| IBIS file stm32u595_599_5a5_5a9_lqfp144_smps.ibs
[IBIS ver] 4.2
[File name] stm32u595_599_5a5_5a9_lqfp144_smps.ibs
[File Rev] rev2.1
[Date]  11-09-2023
[Source] Data Created at STMicroelectronics
[Notes]  File originated from ELDO simulations.
[Disclaimer]  This information is for modeling purpose only and is
   not guaranteed. The information is subject to change without
   notice.
[Copyright] Copyright 2023 STMicroelectronics Inc.
|   Component stm32u595_599_5a5_5a9_lqfp144_smps
[Component] stm32u595_599_5a5_5a9_lqfp144_smps
[Manufacturer] STMicroelectronics
[Package]
| variable   typ   min   max
R_pkg  0  NA  NA
L_pkg  0  NA  NA
C_pkg  0  NA  NA
[Pin]   signal_name   model_name
1  PE2  io8_100m_hslv_ft
2  PE3  io8_100m_hslv_tamp_ft
3  PE4  io8_100m_hslv_tamp_ft
4  PE5  io8_100m_hslv_tamp_ft
5  PE6  io8_100m_hslv_tamp_ft
6  VBAT  power
7  PC13  io8_100m_ft
8  PC14-OSC32_IN  nc
9  PC15-OSC32_OUT  nc
10  PF0  io8_100m_hslv_ft
11  PF1  io8_100m_hslv_ft
12  PF2  io8_100m_hslv_ft
13  PF3  io8_100m_hslv_ft
14  PF4  io8_100m_i2c_ft
15  PF5  io8_100m_i2c_ft
16  VSS  gnd
17  VDD  power
18  PF6  io8_100m_hslv_ft
19  PF7  io8_100m_hslv_ft
20  PF8  io8_100m_hslv_ft
21  PF9  io8_100m_hslv_ft
22  PF10  io8_166m_hslv_ft
23  PH0-OSC_IN  nc
24  PH1-OSC_OUT  nc
25  NRST  nc
26  PC0  io8_100m_hslv_ft
27  PC1  io8_spi_hslv_ft
28  PC2  io8_100m_hslv_ft
29  PC3  io8_100m_hslv_ft
30  VSSA  nc
31  VREFP  nc
32  VDDA  nc
33  PA0  io8_100m_hslv_tamp_ft
34  PA1  io8_100m_hslv_tamp_ft
35  PA2  io8_100m_hslv_ft
36  PA3  io8_166m_hslv_ft
37  VSS  gnd
38  VDD  power
39  PA4  io8_100m_hslv_ft
40  PA5  io8_100m_ft
41  PA6  io8_100m_hslv_ft
42  PA7  io8_100m_hslv_ft
43  PB0  io8_100m_hslv_ft
44  PB1  io8_100m_hslv_ft
45  PB2  io8_100m_hslv_tamp_ft
46  PF11  io8_166m_hslv_ft
47  PF12  io8_100m_hslv_ft
48  VSS  gnd
49  VDD  power
50  PF13  io8_100m_hslv_ft
51  PF14  io8_100m_hslv_ft
52  PF15  io8_100m_hslv_ft
53  PG0  io8_100m_hslv_ft
54  PG1  io8_100m_hslv_ft
55  PE7  io8_100m_hslv_ft
56  PE8  io8_100m_hslv_ft
57  PE9  io8_166m_hslv_ft
58  VSS  gnd
59  VDD  power
60  PE10  io8_166m_hslv_ft
61  PE11  io8_100m_hslv_ft
62  PE12  io8_100m_hslv_ft
63  PE13  io8_100m_hslv_ft
64  PE14  io8_100m_hslv_ft
65  PE15  io8_100m_hslv_ft
66  PB10  io8_spi_hslv_ft
67  PB11  io8_100m_hslv_ft
68  VLXSMPS  nc
69  VDDSMPS  nc
70  VSSSMPS  nc
71  VDD11  nc
72  VSS  gnd
73  VDD  power
74  PB13  io8_100m_i2c_ft
75  PB14  io8_100m_i2c_ft
76  PB15  nc
77  PD8  io8_100m_hslv_ft
78  PD9  io8_100m_hslv_ft
79  PD10  io8_100m_hslv_ft
80  PD11  io8_100m_hslv_ft
81  PD12  io8_100m_hslv_ft
82  PD13  io8_100m_hslv_ft
83  VSS  gnd
84  VDD  power
85  PD14  io8_100m_hslv_ft
86  PD15  io8_100m_hslv_ft
87  PG2  io8_100m_hslv_ft
88  PG3  io8_100m_hslv_ft
89  PG4  io8_100m_hslv_ft
90  PG5  io8_100m_hslv_ft
91  PG6  io8_100m_hslv_ft
92  PG7  io8_100m_hslv_ft
93  PG8  io8_100m_i2c_ft
94  VSS  gnd
95  VDDIO2  power
96  PC6  io8_100m_ft
97  PC7  io8_100m_ft
98  PC8  io8_100m_ft
99  PC9  io8_100m_ft
100  PA8  io8_166m_hslv_ft
101  PA9  io8_100m_usb_vbus_ft
102  PA10  io8_100m_usb_id
103  PA11  io8_100m_ft
104  PA12  io8_100m_ft
105  PA13  io8_100m_ft
106  VDDUSB  power
107  VSS  gnd
108  VDD  power
109  PA14  io8_100m_ft
110  PA15  nc
111  PC10  io8_100m_ft
112  PC11  io8_100m_hslv_ft
113  PC12  io8_166m_hslv_ft
114  PD0  io8_100m_hslv_ft
115  PD1  io8_100m_hslv_ft
116  PD2  io8_100m_ft
117  PD3  io8_166m_hslv_ft
118  PD4  io8_100m_hslv_ft
119  PD5  io8_100m_hslv_ft
120  VSS  gnd
121  VDD  power
122  PD6  io8_166m_hslv_ft
123  PD7  io8_100m_hslv_ft
124  PG9  io8_100m_hslv_ft
125  PG10  io8_100m_hslv_ft
126  PG12  io8_100m_hslv_ft
127  PG13  io8_100m_hslv_ft
128  PG14  io8_100m_hslv_ft
129  VSS  gnd
130  VDDIO2  power
131  PG15  io8_100m_hslv_ft
132  PB3  io8_100m_i2c_ft
133  PB4  io8_100m_i2c_ft
134  PB5  io8_166m_hslv_ft
135  PB6  io8_100m_i2c_ft
136  PB7  io8_spi_hslv_ft
137  PH3-BOOT0  nc
138  PB8  io8_100m_i2c_ft
139  PB9  io8_100m_i2c_ft
140  PE0  io8_100m_hslv_ft
141  PE1  io8_100m_hslv_ft
142  VDD11  nc
143  VSS  gnd
144  VDD  power
[Package Model]   481-lqfp-20x20-144-smps-221207
[Pin Mapping]   pulldown_ref   pullup_ref   | Comment
1  gndio  vddiom
2  gndio  vddiom
3  gndio  vddiom
4  gndio  vddiom
5  gndio  vddiom
6  nc  vsw
7  gndio  vddiom  | Depending on IO usage
| 7  gndio  vsw  | Depending on IO usage
8  nc  nc
9  nc  nc
10  gndio  vddiom
11  gndio  vddiom
12  gndio  vddiom
13  gndio  vddiom
14  gndio  vddiom
15  gndio  vddiom
16  gndio  nc
17  nc  vddiom
18  gndio  vddiom
19  gndio  vddiom
20  gndio  vddiom
21  gndio  vddiom
22  gndio  vddiom
23  nc  nc
24  nc  nc
25  nc  nc
26  gndio  vddiom
27  gndio  vddiom
28  gndio  vddiom
29  gndio  vddiom
30  nc  nc
31  nc  nc
32  nc  nc
33  gndio  vddiom
34  gndio  vddiom
35  gndio  vddiom
36  gndio  vddiom
37  gndio  nc
38  nc  vddiom
39  gndio  vddiom
40  gndio  vddiom
41  gndio  vddiom
42  gndio  vddiom
43  gndio  vddiom
44  gndio  vddiom
45  gndio  vddiom
46  gndio  vddiom
47  gndio  vddiom
48  gndio  nc
49  nc  vddiom
50  gndio  vddiom
51  gndio  vddiom
52  gndio  vddiom
53  gndio  vddiom
54  gndio  vddiom
55  gndio  vddiom
56  gndio  vddiom
57  gndio  vddiom
58  gndio  nc
59  nc  vddiom
60  gndio  vddiom
61  gndio  vddiom
62  gndio  vddiom
63  gndio  vddiom
64  gndio  vddiom
65  gndio  vddiom
66  gndio  vddiom
67  gndio  vddiom
68  nc  nc
69  nc  nc
70  nc  nc
71  nc  nc
72  gndio  nc
73  nc  vddiom
74  gndio  vddiom
75  gndio  vddiom
76  nc  nc
77  gndio  vddiom
78  gndio  vddiom
79  gndio  vddiom
80  gndio  vddiom
81  gndio  vddiom
82  gndio  vddiom
83  gndio  nc
84  nc  vddiom
85  gndio  vddiom
86  gndio  vddiom
87  gndio  vddiom  | Depending on IO usage
| 87  gndio  vddio2  | Depending on IO usage
88  gndio  vddiom  | Depending on IO usage
| 88  gndio  vddio2  | Depending on IO usage
89  gndio  vddiom  | Depending on IO usage
| 89  gndio  vddio2  | Depending on IO usage
90  gndio  vddiom  | Depending on IO usage
| 90  gndio  vddio2  | Depending on IO usage
91  gndio  vddiom  | Depending on IO usage
| 91  gndio  vddio2  | Depending on IO usage
92  gndio  vddiom  | Depending on IO usage
| 92  gndio  vddio2  | Depending on IO usage
93  gndio  vddiom  | Depending on IO usage
| 93  gndio  vddio2  | Depending on IO usage
94  gndio  nc
95  nc  vddio2
96  gndio  vddiom
97  gndio  vddiom
98  gndio  vddiom
99  gndio  vddiom
100  gndio  vddiom
101  gndio  vddiom  | Depending on IO usage
| 101  gndio  vddusb  | Depending on IO usage
102  gndio  vddiom  | Depending on IO usage
| 102  gndio  vddusb  | Depending on IO usage
103  gndio  vddiom  | Depending on IO usage
| 103  gndio  vddusb  | Depending on IO usage
104  gndio  vddiom  | Depending on IO usage
| 104  gndio  vddusb  | Depending on IO usage
105  gndio  vddiom  | Depending on IO usage
| 105  gndio  vddusb  | Depending on IO usage
106  nc  vddusb
107  gndio  nc
108  nc  vddiom
109  gndio  vddiom
110  nc  nc
111  gndio  vddiom
112  gndio  vddiom
113  gndio  vddiom
114  gndio  vddiom
115  gndio  vddiom
116  gndio  vddiom
117  gndio  vddiom
118  gndio  vddiom
119  gndio  vddiom
120  gndio  nc
121  nc  vddiom
122  gndio  vddiom
123  gndio  vddiom
124  gndio  vddiom  | Depending on IO usage
| 124  gndio  vddio2  | Depending on IO usage
125  gndio  vddiom  | Depending on IO usage
| 125  gndio  vddio2  | Depending on IO usage
126  gndio  vddiom  | Depending on IO usage
| 126  gndio  vddio2  | Depending on IO usage
127  gndio  vddiom  | Depending on IO usage
| 127  gndio  vddio2  | Depending on IO usage
128  gndio  vddiom  | Depending on IO usage
| 128  gndio  vddio2  | Depending on IO usage
129  gndio  nc
130  nc  vddio2
131  gndio  vddiom  | Depending on IO usage
| 131  gndio  vddio2  | Depending on IO usage
132  gndio  vddiom
133  gndio  vddiom
134  gndio  vddiom
135  gndio  vddiom
136  gndio  vddiom
137  nc  nc
138  gndio  vddiom
139  gndio  vddiom
140  gndio  vddiom
141  gndio  vddiom
142  nc  nc
143  gndio  nc
144  nc  vddiom
[Model Selector] io8_100m_ft
io8_100m_ft_hs_1v2  "IO8_FT 100MHz high speed @ 1.2V"
io8_100m_ft_fs_1v2  "IO8_FT 100MHz fast speed @ 1.2V"
io8_100m_ft_fs_pd_1v2  "IO8_FT 100MHz fast speed @ 1.2V pulldown"
io8_100m_ft_ms_1v2  "IO8_FT 100MHz med speed @ 1.2V"
io8_100m_ft_ms_pd_1v2  "IO8_FT 100MHz med speed @ 1.2V pulldown"
io8_100m_ft_ls_1v2  "IO8_FT 100MHz low speed @ 1.2V"
io8_100m_ft_ls_pd_1v2  "IO8_FT 100MHz low speed @ 1.2V pulldown"
io8_100m_ft_hs_1v8  "IO8_FT 100MHz high speed @ 1.8V"
io8_100m_ft_hs_pd_1v8  "IO8_FT 100MHz high speed @ 1.8V pulldown"
io8_100m_ft_fs_1v8  "IO8_FT 100MHz fast speed @ 1.8V"
io8_100m_ft_fs_pd_1v8  "IO8_FT 100MHz fast speed @ 1.8V pulldown"
io8_100m_ft_ms_1v8  "IO8_FT 100MHz med speed @ 1.8V"
io8_100m_ft_ms_pd_1v8  "IO8_FT 100MHz med speed @ 1.8V pulldown"
io8_100m_ft_ls_1v8  "IO8_FT 100MHz low speed @ 1.8V"
io8_100m_ft_ls_pd_1v8  "IO8_FT 100MHz low speed @ 1.8V pulldown"
io8_100m_ft_hs_3v3  "IO8_FT 100MHz high speed @ 3.3V"
io8_100m_ft_hs_pd_3v3  "IO8_FT 100MHz high speed @ 3.3V pulldown"
io8_100m_ft_fs_3v3  "IO8_FT 100MHz fast speed @ 3.3V"
io8_100m_ft_fs_pd_3v3  "IO8_FT 100MHz fast speed @ 3.3V pulldown"
io8_100m_ft_ms_3v3  "IO8_FT 100MHz med speed @ 3.3V"
io8_100m_ft_ms_pd_3v3  "IO8_FT 100MHz med speed @ 3.3V pulldown"
io8_100m_ft_ls_3v3  "IO8_FT 100MHz low speed @ 3.3V"
io8_100m_ft_ls_pd_3v3  "IO8_FT 100MHz low speed @ 3.3V pulldown"
[Model Selector] io8_100m_hslv_ft
io8_100m_ft_hs_1v2  "IO8_FT 100MHz high speed @ 1.2V"
io8_100m_ft_hs_pu_1v2  "IO8_FT 100MHz high speed @ 1.2V pullup"
io8_100m_ft_hs_pd_1v2  "IO8_FT 100MHz high speed @ 1.2V pulldown"
io8_100m_ft_fs_1v2  "IO8_FT 100MHz fast speed @ 1.2V"
io8_100m_ft_fs_pu_1v2  "IO8_FT 100MHz fast speed @ 1.2V pullup"
io8_100m_ft_fs_pd_1v2  "IO8_FT 100MHz fast speed @ 1.2V pulldown"
io8_100m_ft_ms_1v2  "IO8_FT 100MHz med speed @ 1.2V"
io8_100m_ft_ms_pu_1v2  "IO8_FT 100MHz med speed @ 1.2V pullup"
io8_100m_ft_ms_pd_1v2  "IO8_FT 100MHz med speed @ 1.2V pulldown"
io8_100m_ft_ls_1v2  "IO8_FT 100MHz low speed @ 1.2V"
io8_100m_ft_ls_pu_1v2  "IO8_FT 100MHz low speed @ 1.2V pullup"
io8_100m_ft_ls_pd_1v2  "IO8_FT 100MHz low speed @ 1.2V pulldown"
io8_100m_ft_hs_1v8  "IO8_FT 100MHz high speed @ 1.8V"
io8_100m_ft_hs_pu_1v8  "IO8_FT 100MHz high speed @ 1.8V pullup"
io8_100m_ft_hs_pd_1v8  "IO8_FT 100MHz high speed @ 1.8V pulldown"
io8_100m_ft_fs_1v8  "IO8_FT 100MHz fast speed @ 1.8V"
io8_100m_ft_fs_pu_1v8  "IO8_FT 100MHz fast speed @ 1.8V pullup"
io8_100m_ft_fs_pd_1v8  "IO8_FT 100MHz fast speed @ 1.8V pulldown"
io8_100m_ft_ms_1v8  "IO8_FT 100MHz med speed @ 1.8V"
io8_100m_ft_ms_pu_1v8  "IO8_FT 100MHz med speed @ 1.8V pullup"
io8_100m_ft_ms_pd_1v8  "IO8_FT 100MHz med speed @ 1.8V pulldown"
io8_100m_ft_ls_1v8  "IO8_FT 100MHz low speed @ 1.8V"
io8_100m_ft_ls_pu_1v8  "IO8_FT 100MHz low speed @ 1.8V pullup"
io8_100m_ft_ls_pd_1v8  "IO8_FT 100MHz low speed @ 1.8V pulldown"
io8_100m_ft_hs_3v3  "IO8_FT 100MHz high speed @ 3.3V"
io8_100m_ft_hs_pu_3v3  "IO8_FT 100MHz high speed @ 3.3V pullup"
io8_100m_ft_hs_pd_3v3  "IO8_FT 100MHz high speed @ 3.3V pulldown"
io8_100m_ft_fs_3v3  "IO8_FT 100MHz fast speed @ 3.3V"
io8_100m_ft_fs_pu_3v3  "IO8_FT 100MHz fast speed @ 3.3V pullup"
io8_100m_ft_fs_pd_3v3  "IO8_FT 100MHz fast speed @ 3.3V pulldown"
io8_100m_ft_ms_3v3  "IO8_FT 100MHz med speed @ 3.3V"
io8_100m_ft_ms_pu_3v3  "IO8_FT 100MHz med speed @ 3.3V pullup"
io8_100m_ft_ms_pd_3v3  "IO8_FT 100MHz med speed @ 3.3V pulldown"
io8_100m_ft_ls_3v3  "IO8_FT 100MHz low speed @ 3.3V"
io8_100m_ft_ls_pu_3v3  "IO8_FT 100MHz low speed @ 3.3V pullup"
io8_100m_ft_ls_pd_3v3  "IO8_FT 100MHz low speed @ 3.3V pulldown"
io8_100m_hslv_ft_hs_1v2  "IO8_FT 100MHz HSLV high speed @ 1.2V"
io8_100m_hslv_ft_hs_pu_1v2  "IO8_FT 100MHz HSLV high speed @ 1.2V pullup"
io8_100m_hslv_ft_hs_pd_1v2  "IO8_FT 100MHz HSLV high speed @ 1.2V pulldown"
io8_100m_hslv_ft_fs_1v2  "IO8_FT 100MHz HSLV fast speed @ 1.2V"
io8_100m_hslv_ft_fs_pu_1v2  "IO8_FT 100MHz HSLV fast speed @ 1.2V pullup"
io8_100m_hslv_ft_fs_pd_1v2  "IO8_FT 100MHz HSLV fast speed @ 1.2V pulldown"
io8_100m_hslv_ft_ms_1v2  "IO8_FT 100MHz HSLV med speed @ 1.2V"
io8_100m_hslv_ft_ms_pu_1v2  "IO8_FT 100MHz HSLV med speed @ 1.2V pullup"
io8_100m_hslv_ft_ms_pd_1v2  "IO8_FT 100MHz HSLV med speed @ 1.2V pulldown"
io8_100m_hslv_ft_ls_1v2  "IO8_FT 100MHz HSLV low speed @ 1.2V"
io8_100m_hslv_ft_ls_pu_1v2  "IO8_FT 100MHz HSLV low speed @ 1.2V pullup"
io8_100m_hslv_ft_ls_pd_1v2  "IO8_FT 100MHz HSLV low speed @ 1.2V pulldown"
io8_100m_hslv_ft_hs_1v8  "IO8_FT 100MHz HSLV high speed @ 1.8V"
io8_100m_hslv_ft_hs_pu_1v8  "IO8_FT 100MHz HSLV high speed @ 1.8V pullup"
io8_100m_hslv_ft_hs_pd_1v8  "IO8_FT 100MHz HSLV high speed @ 1.8V pulldown"
io8_100m_hslv_ft_fs_1v8  "IO8_FT 100MHz HSLV fast speed @ 1.8V"
io8_100m_hslv_ft_fs_pu_1v8  "IO8_FT 100MHz HSLV fast speed @ 1.8V pullup"
io8_100m_hslv_ft_fs_pd_1v8  "IO8_FT 100MHz HSLV fast speed @ 1.8V pulldown"
io8_100m_hslv_ft_ms_1v8  "IO8_FT 100MHz HSLV med speed @ 1.8V"
io8_100m_hslv_ft_ms_pu_1v8  "IO8_FT 100MHz HSLV med speed @ 1.8V pullup"
io8_100m_hslv_ft_ms_pd_1v8  "IO8_FT 100MHz HSLV med speed @ 1.8V pulldown"
io8_100m_hslv_ft_ls_1v8  "IO8_FT 100MHz HSLV low speed @ 1.8V"
io8_100m_hslv_ft_ls_pu_1v8  "IO8_FT 100MHz HSLV low speed @ 1.8V pullup"
io8_100m_hslv_ft_ls_pd_1v8  "IO8_FT 100MHz HSLV low speed @ 1.8V pulldown"
io8_100m_hslv_ft_hs_2v5  "IO8_FT 100MHz HSLV high speed @ 2.5V"
io8_100m_hslv_ft_hs_pu_2v5  "IO8_FT 100MHz HSLV high speed @ 2.5V pullup"
io8_100m_hslv_ft_hs_pd_2v5  "IO8_FT 100MHz HSLV high speed @ 2.5V pulldown"
io8_100m_hslv_ft_fs_2v5  "IO8_FT 100MHz HSLV fast speed @ 2.5V"
io8_100m_hslv_ft_fs_pu_2v5  "IO8_FT 100MHz HSLV fast speed @ 2.5V pullup"
io8_100m_hslv_ft_fs_pd_2v5  "IO8_FT 100MHz HSLV fast speed @ 2.5V pulldown"
io8_100m_hslv_ft_ms_2v5  "IO8_FT 100MHz HSLV med speed @ 2.5V"
io8_100m_hslv_ft_ms_pu_2v5  "IO8_FT 100MHz HSLV med speed @ 2.5V pullup"
io8_100m_hslv_ft_ms_pd_2v5  "IO8_FT 100MHz HSLV med speed @ 2.5V pulldown"
io8_100m_hslv_ft_ls_2v5  "IO8_FT 100MHz HSLV low speed @ 2.5V"
io8_100m_hslv_ft_ls_pu_2v5  "IO8_FT 100MHz HSLV low speed @ 2.5V pullup"
io8_100m_hslv_ft_ls_pd_2v5  "IO8_FT 100MHz HSLV low speed @ 2.5V pulldown"
[Model Selector] io8_100m_hslv_tamp_ft
io8_100m_ft_hs_1v2  "IO8_FT 100MHz high speed @ 1.2V"
io8_100m_ft_hs_pu_1v2  "IO8_FT 100MHz high speed @ 1.2V pullup"
io8_100m_ft_hs_pd_1v2  "IO8_FT 100MHz high speed @ 1.2V pulldown"
io8_100m_ft_fs_1v2  "IO8_FT 100MHz fast speed @ 1.2V"
io8_100m_ft_fs_pu_1v2  "IO8_FT 100MHz fast speed @ 1.2V pullup"
io8_100m_ft_fs_pd_1v2  "IO8_FT 100MHz fast speed @ 1.2V pulldown"
io8_100m_ft_ms_1v2  "IO8_FT 100MHz med speed @ 1.2V"
io8_100m_ft_ms_pu_1v2  "IO8_FT 100MHz med speed @ 1.2V pullup"
io8_100m_ft_ms_pd_1v2  "IO8_FT 100MHz med speed @ 1.2V pulldown"
io8_100m_ft_ls_1v2  "IO8_FT 100MHz low speed @ 1.2V"
io8_100m_ft_ls_pu_1v2  "IO8_FT 100MHz low speed @ 1.2V pullup"
io8_100m_ft_ls_pd_1v2  "IO8_FT 100MHz low speed @ 1.2V pulldown"
io8_100m_ft_hs_1v8  "IO8_FT 100MHz high speed @ 1.8V"
io8_100m_ft_hs_pu_1v8  "IO8_FT 100MHz high speed @ 1.8V pullup"
io8_100m_ft_hs_pd_1v8  "IO8_FT 100MHz high speed @ 1.8V pulldown"
io8_100m_ft_fs_1v8  "IO8_FT 100MHz fast speed @ 1.8V"
io8_100m_ft_fs_pu_1v8  "IO8_FT 100MHz fast speed @ 1.8V pullup"
io8_100m_ft_fs_pd_1v8  "IO8_FT 100MHz fast speed @ 1.8V pulldown"
io8_100m_ft_ms_1v8  "IO8_FT 100MHz med speed @ 1.8V"
io8_100m_ft_ms_pu_1v8  "IO8_FT 100MHz med speed @ 1.8V pullup"
io8_100m_ft_ms_pd_1v8  "IO8_FT 100MHz med speed @ 1.8V pulldown"
io8_100m_ft_ls_1v8  "IO8_FT 100MHz low speed @ 1.8V"
io8_100m_ft_ls_pu_1v8  "IO8_FT 100MHz low speed @ 1.8V pullup"
io8_100m_ft_ls_pd_1v8  "IO8_FT 100MHz low speed @ 1.8V pulldown"
io8_100m_ft_hs_3v3  "IO8_FT 100MHz high speed @ 3.3V"
io8_100m_ft_hs_pu_3v3  "IO8_FT 100MHz high speed @ 3.3V pullup"
io8_100m_ft_hs_pd_3v3  "IO8_FT 100MHz high speed @ 3.3V pulldown"
io8_100m_ft_fs_3v3  "IO8_FT 100MHz fast speed @ 3.3V"
io8_100m_ft_fs_pu_3v3  "IO8_FT 100MHz fast speed @ 3.3V pullup"
io8_100m_ft_fs_pd_3v3  "IO8_FT 100MHz fast speed @ 3.3V pulldown"
io8_100m_ft_ms_3v3  "IO8_FT 100MHz med speed @ 3.3V"
io8_100m_ft_ms_pu_3v3  "IO8_FT 100MHz med speed @ 3.3V pullup"
io8_100m_ft_ms_pd_3v3  "IO8_FT 100MHz med speed @ 3.3V pulldown"
io8_100m_ft_ls_3v3  "IO8_FT 100MHz low speed @ 3.3V"
io8_100m_ft_ls_pu_3v3  "IO8_FT 100MHz low speed @ 3.3V pullup"
io8_100m_ft_ls_pd_3v3  "IO8_FT 100MHz low speed @ 3.3V pulldown"
io8_100m_hslv_ft_hs_1v2  "IO8_FT 100MHz HSLV high speed @ 1.2V"
io8_100m_hslv_ft_hs_pu_1v2  "IO8_FT 100MHz HSLV high speed @ 1.2V pullup"
io8_100m_hslv_ft_hs_pd_1v2  "IO8_FT 100MHz HSLV high speed @ 1.2V pulldown"
io8_100m_hslv_ft_fs_1v2  "IO8_FT 100MHz HSLV fast speed @ 1.2V"
io8_100m_hslv_ft_fs_pu_1v2  "IO8_FT 100MHz HSLV fast speed @ 1.2V pullup"
io8_100m_hslv_ft_fs_pd_1v2  "IO8_FT 100MHz HSLV fast speed @ 1.2V pulldown"
io8_100m_hslv_ft_ms_1v2  "IO8_FT 100MHz HSLV med speed @ 1.2V"
io8_100m_hslv_ft_ms_pu_1v2  "IO8_FT 100MHz HSLV med speed @ 1.2V pullup"
io8_100m_hslv_ft_ms_pd_1v2  "IO8_FT 100MHz HSLV med speed @ 1.2V pulldown"
io8_100m_hslv_ft_ls_1v2  "IO8_FT 100MHz HSLV low speed @ 1.2V"
io8_100m_hslv_ft_ls_pu_1v2  "IO8_FT 100MHz HSLV low speed @ 1.2V pullup"
io8_100m_hslv_ft_ls_pd_1v2  "IO8_FT 100MHz HSLV low speed @ 1.2V pulldown"
io8_100m_hslv_ft_hs_1v8  "IO8_FT 100MHz HSLV high speed @ 1.8V"
io8_100m_hslv_ft_hs_pu_1v8  "IO8_FT 100MHz HSLV high speed @ 1.8V pullup"
io8_100m_hslv_ft_hs_pd_1v8  "IO8_FT 100MHz HSLV high speed @ 1.8V pulldown"
io8_100m_hslv_ft_fs_1v8  "IO8_FT 100MHz HSLV fast speed @ 1.8V"
io8_100m_hslv_ft_fs_pu_1v8  "IO8_FT 100MHz HSLV fast speed @ 1.8V pullup"
io8_100m_hslv_ft_fs_pd_1v8  "IO8_FT 100MHz HSLV fast speed @ 1.8V pulldown"
io8_100m_hslv_ft_ms_1v8  "IO8_FT 100MHz HSLV med speed @ 1.8V"
io8_100m_hslv_ft_ms_pu_1v8  "IO8_FT 100MHz HSLV med speed @ 1.8V pullup"
io8_100m_hslv_ft_ms_pd_1v8  "IO8_FT 100MHz HSLV med speed @ 1.8V pulldown"
io8_100m_hslv_ft_ls_1v8  "IO8_FT 100MHz HSLV low speed @ 1.8V"
io8_100m_hslv_ft_ls_pu_1v8  "IO8_FT 100MHz HSLV low speed @ 1.8V pullup"
io8_100m_hslv_ft_ls_pd_1v8  "IO8_FT 100MHz HSLV low speed @ 1.8V pulldown"
io8_100m_hslv_ft_hs_2v5  "IO8_FT 100MHz HSLV high speed @ 2.5V"
io8_100m_hslv_ft_hs_pu_2v5  "IO8_FT 100MHz HSLV high speed @ 2.5V pullup"
io8_100m_hslv_ft_hs_pd_2v5  "IO8_FT 100MHz HSLV high speed @ 2.5V pulldown"
io8_100m_hslv_ft_fs_2v5  "IO8_FT 100MHz HSLV fast speed @ 2.5V"
io8_100m_hslv_ft_fs_pu_2v5  "IO8_FT 100MHz HSLV fast speed @ 2.5V pullup"
io8_100m_hslv_ft_fs_pd_2v5  "IO8_FT 100MHz HSLV fast speed @ 2.5V pulldown"
io8_100m_hslv_ft_ms_2v5  "IO8_FT 100MHz HSLV med speed @ 2.5V"
io8_100m_hslv_ft_ms_pu_2v5  "IO8_FT 100MHz HSLV med speed @ 2.5V pullup"
io8_100m_hslv_ft_ms_pd_2v5  "IO8_FT 100MHz HSLV med speed @ 2.5V pulldown"
io8_100m_hslv_ft_ls_2v5  "IO8_FT 100MHz HSLV low speed @ 2.5V"
io8_100m_hslv_ft_ls_pu_2v5  "IO8_FT 100MHz HSLV low speed @ 2.5V pullup"
io8_100m_hslv_ft_ls_pd_2v5  "IO8_FT 100MHz HSLV low speed @ 2.5V pulldown"
io8_ft_v33_hs_1v2  "IO8_FT_V33 high speed @ 1.2V"
io8_ft_v33_hs_pu_1v2  "IO8_FT_V33 high speed @ 1.2V pullup"
io8_ft_v33_hs_pd_1v2  "IO8_FT_V33 high speed @ 1.2V pulldown"
io8_ft_v33_fs_1v2  "IO8_FT_V33 fast speed @ 1.2V"
io8_ft_v33_fs_pu_1v2  "IO8_FT_V33 fast speed @ 1.2V pullup"
io8_ft_v33_fs_pd_1v2  "IO8_FT_V33 fast speed @ 1.2V pulldown"
io8_ft_v33_ms_1v2  "IO8_FT_V33 med speed @ 1.2V"
io8_ft_v33_ms_pu_1v2  "IO8_FT_V33 med speed @ 1.2V pullup"
io8_ft_v33_ms_pd_1v2  "IO8_FT_V33 med speed @ 1.2V pulldown"
io8_ft_v33_ls_1v2  "IO8_FT_V33 low speed @ 1.2V"
io8_ft_v33_ls_pu_1v2  "IO8_FT_V33 low speed @ 1.2V pullup"
io8_ft_v33_ls_pd_1v2  "IO8_FT_V33 low speed @ 1.2V pulldown"
io8_ft_v33_hs_1v8  "IO8_FT_V33 high speed @ 1.8V"
io8_ft_v33_hs_pu_1v8  "IO8_FT_V33 high speed @ 1.8V pullup"
io8_ft_v33_hs_pd_1v8  "IO8_FT_V33 high speed @ 1.8V pulldown"
io8_ft_v33_fs_1v8  "IO8_FT_V33 fast speed @ 1.8V"
io8_ft_v33_fs_pu_1v8  "IO8_FT_V33 fast speed @ 1.8V pullup"
io8_ft_v33_fs_pd_1v8  "IO8_FT_V33 fast speed @ 1.8V pulldown"
io8_ft_v33_ms_1v8  "IO8_FT_V33 med speed @ 1.8V"
io8_ft_v33_ms_pu_1v8  "IO8_FT_V33 med speed @ 1.8V pullup"
io8_ft_v33_ms_pd_1v8  "IO8_FT_V33 med speed @ 1.8V pulldown"
io8_ft_v33_ls_1v8  "IO8_FT_V33 low speed @ 1.8V"
io8_ft_v33_ls_pu_1v8  "IO8_FT_V33 low speed @ 1.8V pullup"
io8_ft_v33_ls_pd_1v8  "IO8_FT_V33 low speed @ 1.8V pulldown"
io8_ft_v33_hs_3v3  "IO8_FT_V33 high speed @ 3.3V"
io8_ft_v33_hs_pu_3v3  "IO8_FT_V33 high speed @ 3.3V pullup"
io8_ft_v33_hs_pd_3v3  "IO8_FT_V33 high speed @ 3.3V pulldown"
io8_ft_v33_fs_3v3  "IO8_FT_V33 fast speed @ 3.3V"
io8_ft_v33_fs_pu_3v3  "IO8_FT_V33 fast speed @ 3.3V pullup"
io8_ft_v33_fs_pd_3v3  "IO8_FT_V33 fast speed @ 3.3V pulldown"
io8_ft_v33_ms_3v3  "IO8_FT_V33 med speed @ 3.3V"
io8_ft_v33_ms_pu_3v3  "IO8_FT_V33 med speed @ 3.3V pullup"
io8_ft_v33_ms_pd_3v3  "IO8_FT_V33 med speed @ 3.3V pulldown"
io8_ft_v33_ls_3v3  "IO8_FT_V33 low speed @ 3.3V"
io8_ft_v33_ls_pu_3v3  "IO8_FT_V33 low speed @ 3.3V pullup"
io8_ft_v33_ls_pd_3v3  "IO8_FT_V33 low speed @ 3.3V pulldown"
[Model Selector] io8_100m_i2c_ft
io8_100m_ft_hs_1v2  "IO8_FT 100MHz high speed @ 1.2V"
io8_100m_ft_hs_pu_1v2  "IO8_FT 100MHz high speed @ 1.2V pullup"
io8_100m_ft_hs_pd_1v2  "IO8_FT 100MHz high speed @ 1.2V pulldown"
io8_100m_ft_fs_1v2  "IO8_FT 100MHz fast speed @ 1.2V"
io8_100m_ft_fs_pu_1v2  "IO8_FT 100MHz fast speed @ 1.2V pullup"
io8_100m_ft_fs_pd_1v2  "IO8_FT 100MHz fast speed @ 1.2V pulldown"
io8_100m_ft_ms_1v2  "IO8_FT 100MHz med speed @ 1.2V"
io8_100m_ft_ms_pu_1v2  "IO8_FT 100MHz med speed @ 1.2V pullup"
io8_100m_ft_ms_pd_1v2  "IO8_FT 100MHz med speed @ 1.2V pulldown"
io8_100m_ft_ls_1v2  "IO8_FT 100MHz low speed @ 1.2V"
io8_100m_ft_ls_pu_1v2  "IO8_FT 100MHz low speed @ 1.2V pullup"
io8_100m_ft_ls_pd_1v2  "IO8_FT 100MHz low speed @ 1.2V pulldown"
io8_100m_ft_hs_1v8  "IO8_FT 100MHz high speed @ 1.8V"
io8_100m_ft_hs_pu_1v8  "IO8_FT 100MHz high speed @ 1.8V pullup"
io8_100m_ft_hs_pd_1v8  "IO8_FT 100MHz high speed @ 1.8V pulldown"
io8_100m_ft_fs_1v8  "IO8_FT 100MHz fast speed @ 1.8V"
io8_100m_ft_fs_pu_1v8  "IO8_FT 100MHz fast speed @ 1.8V pullup"
io8_100m_ft_fs_pd_1v8  "IO8_FT 100MHz fast speed @ 1.8V pulldown"
io8_100m_ft_ms_1v8  "IO8_FT 100MHz med speed @ 1.8V"
io8_100m_ft_ms_pu_1v8  "IO8_FT 100MHz med speed @ 1.8V pullup"
io8_100m_ft_ms_pd_1v8  "IO8_FT 100MHz med speed @ 1.8V pulldown"
io8_100m_ft_ls_1v8  "IO8_FT 100MHz low speed @ 1.8V"
io8_100m_ft_ls_pu_1v8  "IO8_FT 100MHz low speed @ 1.8V pullup"
io8_100m_ft_ls_pd_1v8  "IO8_FT 100MHz low speed @ 1.8V pulldown"
io8_100m_ft_hs_3v3  "IO8_FT 100MHz high speed @ 3.3V"
io8_100m_ft_hs_pu_3v3  "IO8_FT 100MHz high speed @ 3.3V pullup"
io8_100m_ft_hs_pd_3v3  "IO8_FT 100MHz high speed @ 3.3V pulldown"
io8_100m_ft_fs_3v3  "IO8_FT 100MHz fast speed @ 3.3V"
io8_100m_ft_fs_pu_3v3  "IO8_FT 100MHz fast speed @ 3.3V pullup"
io8_100m_ft_fs_pd_3v3  "IO8_FT 100MHz fast speed @ 3.3V pulldown"
io8_100m_ft_ms_3v3  "IO8_FT 100MHz med speed @ 3.3V"
io8_100m_ft_ms_pu_3v3  "IO8_FT 100MHz med speed @ 3.3V pullup"
io8_100m_ft_ms_pd_3v3  "IO8_FT 100MHz med speed @ 3.3V pulldown"
io8_100m_ft_ls_3v3  "IO8_FT 100MHz low speed @ 3.3V"
io8_100m_ft_ls_pu_3v3  "IO8_FT 100MHz low speed @ 3.3V pullup"
io8_100m_ft_ls_pd_3v3  "IO8_FT 100MHz low speed @ 3.3V pulldown"
io8_100m_i2c_ft_1v2  "IO8_FT 100MHz I2C @ 1.2V"
io8_100m_i2c_ft_pu_1v2  "IO8_FT 100MHz I2C @ 1.2V pullup"
io8_100m_i2c_ft_pd_1v2  "IO8_FT 100MHz I2C @ 1.2V pulldown"
io8_100m_i2c_ft_1v8  "IO8_FT 100MHz I2C @ 1.8V"
io8_100m_i2c_ft_pu_1v8  "IO8_FT 100MHz I2C @ 1.8V pullup"
io8_100m_i2c_ft_pd_1v8  "IO8_FT 100MHz I2C @ 1,8V pulldown"
io8_100m_i2c_ft_3v3  "IO8_FT 100MHz I2C @ 3.3V"
io8_100m_i2c_ft_pu_3v3  "IO8_FT 100MHz I2C HSLV @ 3.3V pullup"
io8_100m_i2c_ft_pd_3v3  "IO8_FT 100MHz I2C @ 3.3V pulldown"
[Model Selector] io8_100m_usb_id
io8_100m_ft_hs_1v2  "IO8_FT 100MHz high speed @ 1.2V"
io8_100m_ft_hs_pu_1v2  "IO8_FT 100MHz high speed @ 1.2V pullup"
io8_100m_ft_hs_pd_1v2  "IO8_FT 100MHz high speed @ 1.2V pulldown"
io8_100m_ft_fs_1v2  "IO8_FT 100MHz fast speed @ 1.2V"
io8_100m_ft_fs_pu_1v2  "IO8_FT 100MHz fast speed @ 1.2V pullup"
io8_100m_ft_fs_pd_1v2  "IO8_FT 100MHz fast speed @ 1.2V pulldown"
io8_100m_ft_ms_1v2  "IO8_FT 100MHz med speed @ 1.2V"
io8_100m_ft_ms_pu_1v2  "IO8_FT 100MHz med speed @ 1.2V pullup"
io8_100m_ft_ms_pd_1v2  "IO8_FT 100MHz med speed @ 1.2V pulldown"
io8_100m_ft_ls_1v2  "IO8_FT 100MHz low speed @ 1.2V"
io8_100m_ft_ls_pu_1v2  "IO8_FT 100MHz low speed @ 1.2V pullup"
io8_100m_ft_ls_pd_1v2  "IO8_FT 100MHz low speed @ 1.2V pulldown"
io8_100m_ft_hs_1v8  "IO8_FT 100MHz high speed @ 1.8V"
io8_100m_ft_hs_pu_1v8  "IO8_FT 100MHz high speed @ 1.8V pullup"
io8_100m_ft_hs_pd_1v8  "IO8_FT 100MHz high speed @ 1.8V pulldown"
io8_100m_ft_fs_1v8  "IO8_FT 100MHz fast speed @ 1.8V"
io8_100m_ft_fs_pu_1v8  "IO8_FT 100MHz fast speed @ 1.8V pullup"
io8_100m_ft_fs_pd_1v8  "IO8_FT 100MHz fast speed @ 1.8V pulldown"
io8_100m_ft_ms_1v8  "IO8_FT 100MHz med speed @ 1.8V"
io8_100m_ft_ms_pu_1v8  "IO8_FT 100MHz med speed @ 1.8V pullup"
io8_100m_ft_ms_pd_1v8  "IO8_FT 100MHz med speed @ 1.8V pulldown"
io8_100m_ft_ls_1v8  "IO8_FT 100MHz low speed @ 1.8V"
io8_100m_ft_ls_pu_1v8  "IO8_FT 100MHz low speed @ 1.8V pullup"
io8_100m_ft_ls_pd_1v8  "IO8_FT 100MHz low speed @ 1.8V pulldown"
io8_100m_ft_hs_3v3  "IO8_FT 100MHz high speed @ 3.3V"
io8_100m_ft_hs_pu_3v3  "IO8_FT 100MHz high speed @ 3.3V pullup"
io8_100m_ft_hs_pd_3v3  "IO8_FT 100MHz high speed @ 3.3V pulldown"
io8_100m_ft_fs_3v3  "IO8_FT 100MHz fast speed @ 3.3V"
io8_100m_ft_fs_pu_3v3  "IO8_FT 100MHz fast speed @ 3.3V pullup"
io8_100m_ft_fs_pd_3v3  "IO8_FT 100MHz fast speed @ 3.3V pulldown"
io8_100m_ft_ms_3v3  "IO8_FT 100MHz med speed @ 3.3V"
io8_100m_ft_ms_pu_3v3  "IO8_FT 100MHz med speed @ 3.3V pullup"
io8_100m_ft_ms_pd_3v3  "IO8_FT 100MHz med speed @ 3.3V pulldown"
io8_100m_ft_ls_3v3  "IO8_FT 100MHz low speed @ 3.3V"
io8_100m_ft_ls_pu_3v3  "IO8_FT 100MHz low speed @ 3.3V pullup"
io8_100m_ft_ls_pd_3v3  "IO8_FT 100MHz low speed @ 3.3V pulldown"
io8usb_id_nopu  "IOUSB ID @ 3.3V"
io8usb_id_pu  "IOUSB ID @ 3.3V pullup"
[Model Selector] io8_100m_usb_vbus_ft
io8_100m_ft_hs_1v2  "IO8_FT 100MHz high speed @ 1.2V"
io8_100m_ft_hs_pu_1v2  "IO8_FT 100MHz high speed @ 1.2V pullup"
io8_100m_ft_hs_pd_1v2  "IO8_FT 100MHz high speed @ 1.2V pulldown"
io8_100m_ft_fs_1v2  "IO8_FT 100MHz fast speed @ 1.2V"
io8_100m_ft_fs_pu_1v2  "IO8_FT 100MHz fast speed @ 1.2V pullup"
io8_100m_ft_fs_pd_1v2  "IO8_FT 100MHz fast speed @ 1.2V pulldown"
io8_100m_ft_ms_1v2  "IO8_FT 100MHz med speed @ 1.2V"
io8_100m_ft_ms_pu_1v2  "IO8_FT 100MHz med speed @ 1.2V pullup"
io8_100m_ft_ms_pd_1v2  "IO8_FT 100MHz med speed @ 1.2V pulldown"
io8_100m_ft_ls_1v2  "IO8_FT 100MHz low speed @ 1.2V"
io8_100m_ft_ls_pu_1v2  "IO8_FT 100MHz low speed @ 1.2V pullup"
io8_100m_ft_ls_pd_1v2  "IO8_FT 100MHz low speed @ 1.2V pulldown"
io8_100m_ft_hs_1v8  "IO8_FT 100MHz high speed @ 1.8V"
io8_100m_ft_hs_pu_1v8  "IO8_FT 100MHz high speed @ 1.8V pullup"
io8_100m_ft_hs_pd_1v8  "IO8_FT 100MHz high speed @ 1.8V pulldown"
io8_100m_ft_fs_1v8  "IO8_FT 100MHz fast speed @ 1.8V"
io8_100m_ft_fs_pu_1v8  "IO8_FT 100MHz fast speed @ 1.8V pullup"
io8_100m_ft_fs_pd_1v8  "IO8_FT 100MHz fast speed @ 1.8V pulldown"
io8_100m_ft_ms_1v8  "IO8_FT 100MHz med speed @ 1.8V"
io8_100m_ft_ms_pu_1v8  "IO8_FT 100MHz med speed @ 1.8V pullup"
io8_100m_ft_ms_pd_1v8  "IO8_FT 100MHz med speed @ 1.8V pulldown"
io8_100m_ft_ls_1v8  "IO8_FT 100MHz low speed @ 1.8V"
io8_100m_ft_ls_pu_1v8  "IO8_FT 100MHz low speed @ 1.8V pullup"
io8_100m_ft_ls_pd_1v8  "IO8_FT 100MHz low speed @ 1.8V pulldown"
io8_100m_ft_hs_3v3  "IO8_FT 100MHz high speed @ 3.3V"
io8_100m_ft_hs_pu_3v3  "IO8_FT 100MHz high speed @ 3.3V pullup"
io8_100m_ft_hs_pd_3v3  "IO8_FT 100MHz high speed @ 3.3V pulldown"
io8_100m_ft_fs_3v3  "IO8_FT 100MHz fast speed @ 3.3V"
io8_100m_ft_fs_pu_3v3  "IO8_FT 100MHz fast speed @ 3.3V pullup"
io8_100m_ft_fs_pd_3v3  "IO8_FT 100MHz fast speed @ 3.3V pulldown"
io8_100m_ft_ms_3v3  "IO8_FT 100MHz med speed @ 3.3V"
io8_100m_ft_ms_pu_3v3  "IO8_FT 100MHz med speed @ 3.3V pullup"
io8_100m_ft_ms_pd_3v3  "IO8_FT 100MHz med speed @ 3.3V pulldown"
io8_100m_ft_ls_3v3  "IO8_FT 100MHz low speed @ 3.3V"
io8_100m_ft_ls_pu_3v3  "IO8_FT 100MHz low speed @ 3.3V pullup"
io8_100m_ft_ls_pd_3v3  "IO8_FT 100MHz low speed @ 3.3V pulldown"
io8usb_adp "IOUSB ADP @ 3.3V"
io8usb_vbus "IOUSB VBUS @ 3.3V"
[Model Selector] io8_166m_hslv_ft
io8_166m_ft_hs_1v2  "IO8_FT 166MHz high speed @ 1.2V"
io8_166m_ft_hs_pu_1v2  "IO8_FT 166MHz high speed @ 1.2V pullup"
io8_166m_ft_hs_pd_1v2  "IO8_FT 166MHz high speed @ 1.2V pulldown"
io8_166m_ft_fs_1v2  "IO8_FT 166MHz fast speed @ 1.2V"
io8_166m_ft_fs_pu_1v2  "IO8_FT 166MHz fast speed @ 1.2V pullup"
io8_166m_ft_fs_pd_1v2  "IO8_FT 166MHz fast speed @ 1.2V pulldown"
io8_166m_ft_ms_1v2  "IO8_FT 166MHz med speed @ 1.2V"
io8_166m_ft_ms_pu_1v2  "IO8_FT 166MHz med speed @ 1.2V pullup"
io8_166m_ft_ms_pd_1v2  "IO8_FT 166MHz med speed @ 1.2V pulldown"
io8_166m_ft_ls_1v2  "IO8_FT 166MHz low speed @ 1.2V"
io8_166m_ft_ls_pu_1v2  "IO8_FT 166MHz low speed @ 1.2V pullup"
io8_166m_ft_ls_pd_1v2  "IO8_FT 166MHz low speed @ 1.2V pulldown"
io8_166m_ft_hs_1v8  "IO8_FT 166MHz high speed @ 1.8V"
io8_166m_ft_hs_pu_1v8  "IO8_FT 166MHz high speed @ 1.8V pullup"
io8_166m_ft_hs_pd_1v8  "IO8_FT 166MHz high speed @ 1.8V pulldown"
io8_166m_ft_fs_1v8  "IO8_FT 166MHz fast speed @ 1.8V"
io8_166m_ft_fs_pu_1v8  "IO8_FT 166MHz fast speed @ 1.8V pullup"
io8_166m_ft_fs_pd_1v8  "IO8_FT 166MHz fast speed @ 1.8V pulldown"
io8_166m_ft_ms_1v8  "IO8_FT 166MHz med speed @ 1.8V"
io8_166m_ft_ms_pu_1v8  "IO8_FT 166MHz med speed @ 1.8V pullup"
io8_166m_ft_ms_pd_1v8  "IO8_FT 166MHz med speed @ 1.8V pulldown"
io8_166m_ft_ls_1v8  "IO8_FT 166MHz low speed @ 1.8V"
io8_166m_ft_ls_pu_1v8  "IO8_FT 166MHz low speed @ 1.8V pullup"
io8_166m_ft_ls_pd_1v8  "IO8_FT 166MHz low speed @ 1.8V pulldown"
io8_166m_ft_hs_3v3  "IO8_FT 166MHz high speed @ 3.3V"
io8_166m_ft_hs_pu_3v3  "IO8_FT 166MHz high speed @ 3.3V pullup"
io8_166m_ft_hs_pd_3v3  "IO8_FT 166MHz high speed @ 3.3V pulldown"
io8_166m_ft_fs_3v3  "IO8_FT 166MHz fast speed @ 3.3V"
io8_166m_ft_fs_pu_3v3  "IO8_FT 166MHz fast speed @ 3.3V pullup"
io8_166m_ft_fs_pd_3v3  "IO8_FT 166MHz fast speed @ 3.3V pulldown"
io8_166m_ft_ms_3v3  "IO8_FT 166MHz med speed @ 3.3V"
io8_166m_ft_ms_pu_3v3  "IO8_FT 166MHz med speed @ 3.3V pullup"
io8_166m_ft_ms_pd_3v3  "IO8_FT 166MHz med speed @ 3.3V pulldown"
io8_166m_ft_ls_3v3  "IO8_FT 166MHz low speed @ 3.3V"
io8_166m_ft_ls_pu_3v3  "IO8_FT 166MHz low speed @ 3.3V pullup"
io8_166m_ft_ls_pd_3v3  "IO8_FT 166MHz low speed @ 3.3V pulldown"
io8_166m_hslv_ft_hs_1v2  "IO8_FT 166MHz HSLV high speed @ 1.2V"
io8_166m_hslv_ft_hs_pu_1v2  "IO8_FT 166MHz HSLV high speed @ 1.2V pullup"
io8_166m_hslv_ft_hs_pd_1v2  "IO8_FT 166MHz HSLV high speed @ 1.2V pulldown"
io8_166m_hslv_ft_fs_1v2  "IO8_FT 166MHz HSLV fast speed @ 1.2V"
io8_166m_hslv_ft_fs_pu_1v2  "IO8_FT 166MHz HSLV fast speed @ 1.2V pullup"
io8_166m_hslv_ft_fs_pd_1v2  "IO8_FT 166MHz HSLV fast speed @ 1.2V pulldown"
io8_166m_hslv_ft_ms_1v2  "IO8_FT 166MHz HSLV med speed @ 1.2V"
io8_166m_hslv_ft_ms_pu_1v2  "IO8_FT 166MHz HSLV med speed @ 1.2V pullup"
io8_166m_hslv_ft_ms_pd_1v2  "IO8_FT 166MHz HSLV med speed @ 1.2V pulldown"
io8_166m_hslv_ft_ls_1v2  "IO8_FT 166MHz HSLV low speed @ 1.2V"
io8_166m_hslv_ft_ls_pu_1v2  "IO8_FT 166MHz HSLV low speed @ 1.2V pullup"
io8_166m_hslv_ft_ls_pd_1v2  "IO8_FT 166MHz HSLV low speed @ 1.2V pulldown"
io8_166m_hslv_ft_hs_1v8  "IO8_FT 166MHz HSLV high speed @ 1.8V"
io8_166m_hslv_ft_hs_pu_1v8  "IO8_FT 166MHz HSLV high speed @ 1.8V pullup"
io8_166m_hslv_ft_hs_pd_1v8  "IO8_FT 166MHz HSLV high speed @ 1.8V pulldown"
io8_166m_hslv_ft_fs_1v8  "IO8_FT 166MHz HSLV fast speed @ 1.8V"
io8_166m_hslv_ft_fs_pu_1v8  "IO8_FT 166MHz HSLV fast speed @ 1.8V pullup"
io8_166m_hslv_ft_fs_pd_1v8  "IO8_FT 166MHz HSLV fast speed @ 1.8V pulldown"
io8_166m_hslv_ft_ms_1v8  "IO8_FT 166MHz HSLV med speed @ 1.8V"
io8_166m_hslv_ft_ms_pu_1v8  "IO8_FT 166MHz HSLV med speed @ 1.8V pullup"
io8_166m_hslv_ft_ms_pd_1v8  "IO8_FT 166MHz HSLV med speed @ 1.8V pulldown"
io8_166m_hslv_ft_ls_1v8  "IO8_FT 166MHz HSLV low speed @ 1.8V"
io8_166m_hslv_ft_ls_pu_1v8  "IO8_FT 166MHz HSLV low speed @ 1.8V pullup"
io8_166m_hslv_ft_ls_pd_1v8  "IO8_FT 166MHz HSLV low speed @ 1.8V pulldown"
io8_166m_hslv_ft_hs_2v5  "IO8_FT 166MHz HSLV high speed @ 2.5V"
io8_166m_hslv_ft_hs_pu_2v5  "IO8_FT 166MHz HSLV high speed @ 2.5V pullup"
io8_166m_hslv_ft_hs_pd_2v5  "IO8_FT 166MHz HSLV high speed @ 2.5V pulldown"
io8_166m_hslv_ft_fs_2v5  "IO8_FT 166MHz HSLV fast speed @ 2.5V"
io8_166m_hslv_ft_fs_pu_2v5  "IO8_FT 166MHz HSLV fast speed @ 2.5V pullup"
io8_166m_hslv_ft_fs_pd_2v5  "IO8_FT 166MHz HSLV fast speed @ 2.5V pulldown"
io8_166m_hslv_ft_ms_2v5  "IO8_FT 166MHz HSLV med speed @ 2.5V"
io8_166m_hslv_ft_ms_pu_2v5  "IO8_FT 166MHz HSLV med speed @ 2.5V pullup"
io8_166m_hslv_ft_ms_pd_2v5  "IO8_FT 166MHz HSLV med speed @ 2.5V pulldown"
io8_166m_hslv_ft_ls_2v5  "IO8_FT 166MHz HSLV low speed @ 2.5V"
io8_166m_hslv_ft_ls_pu_2v5  "IO8_FT 166MHz HSLV low speed @ 2.5V pullup"
io8_166m_hslv_ft_ls_pd_2v5  "IO8_FT 166MHz HSLV low speed @ 2.5V pulldown"
[Model Selector] io8_spi_hslv_ft
io8_spi_ft_hs_1v2  "IO8_FT SPI high speed @ 1.2V"
io8_spi_ft_hs_pu_1v2  "IO8_FT SPI high speed @ 1.2V pullup"
io8_spi_ft_hs_pd_1v2  "IO8_FT SPI high speed @ 1.2V pulldown"
io8_spi_ft_fs_1v2  "IO8_FT SPI fast speed @ 1.2V"
io8_spi_ft_fs_pu_1v2  "IO8_FT SPI fast speed @ 1.2V pullup"
io8_spi_ft_fs_pd_1v2  "IO8_FT SPI fast speed @ 1.2V pulldown"
io8_spi_ft_ms_1v2  "IO8_FT SPI med speed @ 1.2V"
io8_spi_ft_ms_pu_1v2  "IO8_FT SPI med speed @ 1.2V pullup"
io8_spi_ft_ms_pd_1v2  "IO8_FT SPI med speed @ 1.2V pulldown"
io8_spi_ft_ls_1v2  "IO8_FT SPI low speed @ 1.2V"
io8_spi_ft_ls_pu_1v2  "IO8_FT SPI low speed @ 1.2V pullup"
io8_spi_ft_ls_pd_1v2  "IO8_FT SPI low speed @ 1.2V pulldown"
io8_spi_ft_hs_1v8  "IO8_FT SPI high speed @ 1.8V"
io8_spi_ft_hs_pu_1v8  "IO8_FT SPI high speed @ 1.8V pullup"
io8_spi_ft_hs_pd_1v8  "IO8_FT SPI high speed @ 1.8V pulldown"
io8_spi_ft_fs_1v8  "IO8_FT SPI fast speed @ 1.8V"
io8_spi_ft_fs_pu_1v8  "IO8_FT SPI fast speed @ 1.8V pullup"
io8_spi_ft_fs_pd_1v8  "IO8_FT SPI fast speed @ 1.8V pulldown"
io8_spi_ft_ms_1v8  "IO8_FT SPI med speed @ 1.8V"
io8_spi_ft_ms_pu_1v8  "IO8_FT SPI med speed @ 1.8V pullup"
io8_spi_ft_ms_pd_1v8  "IO8_FT SPI med speed @ 1.8V pulldown"
io8_spi_ft_ls_1v8  "IO8_FT SPI low speed @ 1.8V"
io8_spi_ft_ls_pu_1v8  "IO8_FT SPI low speed @ 1.8V pullup"
io8_spi_ft_ls_pd_1v8  "IO8_FT SPI low speed @ 1.8V pulldown"
io8_spi_ft_hs_3v3  "IO8_FT SPI high speed @ 3.3V"
io8_spi_ft_hs_pu_3v3  "IO8_FT SPI high speed @ 3.3V pullup"
io8_spi_ft_hs_pd_3v3  "IO8_FT SPI high speed @ 3.3V pulldown"
io8_spi_ft_fs_3v3  "IO8_FT SPI fast speed @ 3.3V"
io8_spi_ft_fs_pu_3v3  "IO8_FT SPI fast speed @ 3.3V pullup"
io8_spi_ft_fs_pd_3v3  "IO8_FT SPI fast speed @ 3.3V pulldown"
io8_spi_ft_ms_3v3  "IO8_FT SPI med speed @ 3.3V"
io8_spi_ft_ms_pu_3v3  "IO8_FT SPI med speed @ 1.8V pullup"
io8_spi_ft_ms_pd_3v3  "IO8_FT SPI med speed @ 3.3V pulldown"
io8_spi_ft_ls_3v3  "IO8_FT SPI low speed @ 3.3V"
io8_spi_ft_ls_pu_3v3  "IO8_FT SPI low speed @ 3.3V pullup"
io8_spi_ft_ls_pd_3v3  "IO8_FT SPI low speed @ 3.3V pulldown"
io8_spi_hslv_ft_hs_1v2  "IO8_FT SPI HSLV high speed @ 1.2V"
io8_spi_hslv_ft_hs_pu_1v2  "IO8_FT SPI HSLV high speed @ 1.2V pullup"
io8_spi_hslv_ft_hs_pd_1v2  "IO8_FT SPI HSLV high speed @ 1.2V pulldown"
io8_spi_hslv_ft_fs_1v2  "IO8_FT SPI HSLV fast speed @ 1.2V"
io8_spi_hslv_ft_fs_pu_1v2  "IO8_FT SPI HSLV fast speed @ 1.2V pullup"
io8_spi_hslv_ft_fs_pd_1v2  "IO8_FT SPI HSLV fast speed @ 1.2V pulldown"
io8_spi_hslv_ft_ms_1v2  "IO8_FT SPI HSLV med speed @ 1.2V"
io8_spi_hslv_ft_ms_pu_1v2  "IO8_FT SPI HSLV med speed @ 1.2V pullup"
io8_spi_hslv_ft_ms_pd_1v2  "IO8_FT SPI HSLV med speed @ 1.2V pulldown"
io8_spi_hslv_ft_ls_1v2  "IO8_FT SPI HSLV low speed @ 1.2V"
io8_spi_hslv_ft_ls_pu_1v2  "IO8_FT SPI HSLV low speed @ 1.2V pullup"
io8_spi_hslv_ft_ls_pd_1v2  "IO8_FT SPI HSLV low speed @ 1.2V pulldown"
io8_spi_hslv_ft_hs_1v8  "IO8_FT SPI HSLV high speed @ 1.8V"
io8_spi_hslv_ft_hs_pu_1v8  "IO8_FT SPI HSLV high speed @ 1.8V pullup"
io8_spi_hslv_ft_hs_pd_1v8  "IO8_FT SPI HSLV high speed @ 1.8V pulldown"
io8_spi_hslv_ft_fs_1v8  "IO8_FT SPI HSLV fast speed @ 1.8V"
io8_spi_hslv_ft_fs_pu_1v8  "IO8_FT SPI HSLV fast speed @ 1.8V pullup"
io8_spi_hslv_ft_fs_pd_1v8  "IO8_FT SPI HSLV fast speed @ 1.8V pulldown"
io8_spi_hslv_ft_ms_1v8  "IO8_FT SPI HSLV med speed @ 1.8V"
io8_spi_hslv_ft_ms_pu_1v8  "IO8_FT SPI HSLV med speed @ 1.8V pullup"
io8_spi_hslv_ft_ms_pd_1v8  "IO8_FT SPI HSLV med speed @ 1.8V pulldown"
io8_spi_hslv_ft_ls_1v8  "IO8_FT SPI HSLV low speed @ 1.8V"
io8_spi_hslv_ft_ls_pu_1v8  "IO8_FT SPI HSLV low speed @ 1.8V pullup"
io8_spi_hslv_ft_ls_pd_1v8  "IO8_FT SPI HSLV low speed @ 1.8V pulldown"
io8_spi_hslv_ft_hs_2v5  "IO8_FT SPI HSLV high speed @ 2.5V"
io8_spi_hslv_ft_hs_pu_2v5  "IO8_FT SPI HSLV high speed @ 2.5V pullup"
io8_spi_hslv_ft_hs_pd_2v5  "IO8_FT SPI HSLV high speed @ 2.5V pulldown"
io8_spi_hslv_ft_fs_2v5  "IO8_FT SPI HSLV fast speed @ 2.5V"
io8_spi_hslv_ft_fs_pu_2v5  "IO8_FT SPI HSLV fast speed @ 2.5V pullup"
io8_spi_hslv_ft_fs_pd_2v5  "IO8_FT SPI HSLV fast speed @ 2.5V pulldown"
io8_spi_hslv_ft_ms_2v5  "IO8_FT SPI HSLV med speed @ 2.5V"
io8_spi_hslv_ft_ms_pu_2v5  "IO8_FT SPI HSLV med speed @ 2.5V pullup"
io8_spi_hslv_ft_ms_pd_2v5  "IO8_FT SPI HSLV med speed @ 2.5V pulldown"
io8_spi_hslv_ft_ls_2v5  "IO8_FT SPI HSLV low speed @ 2.5V"
io8_spi_hslv_ft_ls_pu_2v5  "IO8_FT SPI HSLV low speed @ 2.5V pullup"
io8_spi_hslv_ft_ls_pd_2v5  "IO8_FT SPI HSLV low speed @ 2.5V pulldown"
[Define Package Model]  481-lqfp-20x20-144-smps-221207
[Manufacturer]  Unknown
[OEM]  Unknown
[Description]  None
[Number Of Pins]  136
[Pin Numbers]
| Pin Num   Terminal Name
25 | NRST
33 | PA0
102 | PA10
103 | PA11
104 | PA12
105 | PA13
109 | PA14
110 | PA15
34 | PA1
35 | PA2
36 | PA3
39 | PA4
40 | PA5
41 | PA6
42 | PA7
100 | PA8
101 | PA9
43 | PB0
66 | PB10
67 | PB11
74 | PB13
75 | PB14
76 | PB15
44 | PB1
45 | PB2
132 | PB3
133 | PB4
134 | PB5
135 | PB6
136 | PB7
138 | PB8
139 | PB9
26 | PC0
111 | PC10
112 | PC11
113 | PC12
7 | PC13
8 | PC14-OSC32_IN
9 | PC15-OSC32_OUT
27 | PC1
28 | PC2
29 | PC3
96 | PC6
97 | PC7
98 | PC8
99 | PC9
114 | PD0
79 | PD10
80 | PD11
81 | PD12
82 | PD13
85 | PD14
86 | PD15
115 | PD1
116 | PD2
117 | PD3
118 | PD4
119 | PD5
122 | PD6
123 | PD7
77 | PD8
78 | PD9
140 | PE0
60 | PE10
61 | PE11
62 | PE12
63 | PE13
64 | PE14
65 | PE15
141 | PE1
1 | PE2
2 | PE3
3 | PE4
4 | PE5
5 | PE6
55 | PE7
56 | PE8
57 | PE9
10 | PF0
22 | PF10
46 | PF11
47 | PF12
50 | PF13
51 | PF14
52 | PF15
11 | PF1
12 | PF2
13 | PF3
14 | PF4
15 | PF5
18 | PF6
19 | PF7
20 | PF8
21 | PF9
53 | PG0
125 | PG10
126 | PG12
127 | PG13
128 | PG14
131 | PG15
54 | PG1
87 | PG2
88 | PG3
89 | PG4
90 | PG5
91 | PG6
92 | PG7
93 | PG8
124 | PG9
23 | PH0-OSC_IN
24 | PH1-OSC_OUT
137 |PH3-BOOT0
142 | VDD11
6 | VBAT
73 | VDD
108 | VDD
144 | VDD
38 | VDD
17 | VDD
49 | VDD
59 | VDD
84 | VDD
121 | VDD
71 | VDD11
106 | VDDUSB
32 | VDDA
95 | VDDIO2
130 | VDDIO2
69 | VDDSMPS
68 | VLXSMPS
31 | VREFP
16 | VSS
30 | VSSA
94 | VSS
129 | VSS
70 | VSSSMPS
|[Merged Pins]  16
|37  |  VSS
|48  |  VSS
|58  |  VSS
|72  |  VSS
|83  |  VSS
|107  |  VSS
|120  |  VSS
|143  |  VSS
[Model Data]
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[End Model Data]
[End Package Model]
| Models and submodels in the file (265): io8_100m_ft_hs_1v2 (I/O), io8_100m_ft_hs_pu_1v2 (I/O), io8_100m_ft_hs_pd_1v2 (I/O), io8_100m_ft_fs_1v2 (I/O), io8_100m_ft_fs_pu_1v2 (I/O), io8_100m_ft_fs_pd_1v2 (I/O), io8_100m_ft_ms_1v2 (I/O), io8_100m_ft_ms_pu_1v2 (I/O), io8_100m_ft_ms_pd_1v2 (I/O), io8_100m_ft_ls_1v2 (I/O), io8_100m_ft_ls_pu_1v2 (I/O), io8_100m_ft_ls_pd_1v2 (I/O), io8_100m_ft_hs_1v8 (I/O), io8_100m_ft_hs_pu_1v8 (I/O), io8_100m_ft_hs_pd_1v8 (I/O), io8_100m_ft_fs_1v8 (I/O), io8_100m_ft_fs_pu_1v8 (I/O), io8_100m_ft_fs_pd_1v8 (I/O), io8_100m_ft_ms_1v8 (I/O), io8_100m_ft_ms_pu_1v8 (I/O), io8_100m_ft_ms_pd_1v8 (I/O), io8_100m_ft_ls_1v8 (I/O), io8_100m_ft_ls_pu_1v8 (I/O), io8_100m_ft_ls_pd_1v8 (I/O), io8_100m_ft_hs_3v3 (I/O), io8_100m_ft_hs_pu_3v3 (I/O), io8_100m_ft_hs_pd_3v3 (I/O), io8_100m_ft_fs_3v3 (I/O), io8_100m_ft_fs_pu_3v3 (I/O), io8_100m_ft_fs_pd_3v3 (I/O), io8_100m_ft_ms_3v3 (I/O), io8_100m_ft_ms_pu_3v3 (I/O), io8_100m_ft_ms_pd_3v3 (I/O), io8_100m_ft_ls_3v3 (I/O), io8_100m_ft_ls_pu_3v3 (I/O), io8_100m_ft_ls_pd_3v3 (I/O), io8_100m_hslv_ft_hs_1v2 (I/O), io8_100m_hslv_ft_hs_pu_1v2 (I/O), io8_100m_hslv_ft_hs_pd_1v2 (I/O), io8_100m_hslv_ft_fs_1v2 (I/O), io8_100m_hslv_ft_fs_pu_1v2 (I/O), io8_100m_hslv_ft_fs_pd_1v2 (I/O), io8_100m_hslv_ft_ms_1v2 (I/O), io8_100m_hslv_ft_ms_pu_1v2 (I/O), io8_100m_hslv_ft_ms_pd_1v2 (I/O), io8_100m_hslv_ft_ls_1v2 (I/O), io8_100m_hslv_ft_ls_pu_1v2 (I/O), io8_100m_hslv_ft_ls_pd_1v2 (I/O), io8_100m_hslv_ft_hs_1v8 (I/O), io8_100m_hslv_ft_hs_pu_1v8 (I/O), io8_100m_hslv_ft_hs_pd_1v8 (I/O), io8_100m_hslv_ft_fs_1v8 (I/O), io8_100m_hslv_ft_fs_pu_1v8 (I/O), io8_100m_hslv_ft_fs_pd_1v8 (I/O), io8_100m_hslv_ft_ms_1v8 (I/O), io8_100m_hslv_ft_ms_pu_1v8 (I/O), io8_100m_hslv_ft_ms_pd_1v8 (I/O), io8_100m_hslv_ft_ls_1v8 (I/O), io8_100m_hslv_ft_ls_pu_1v8 (I/O), io8_100m_hslv_ft_ls_pd_1v8 (I/O), io8_100m_hslv_ft_hs_2v5 (I/O), io8_100m_hslv_ft_hs_pu_2v5 (I/O), io8_100m_hslv_ft_hs_pd_2v5 (I/O), io8_100m_hslv_ft_fs_2v5 (I/O), io8_100m_hslv_ft_fs_pu_2v5 (I/O), io8_100m_hslv_ft_fs_pd_2v5 (I/O), io8_100m_hslv_ft_ms_2v5 (I/O), io8_100m_hslv_ft_ms_pu_2v5 (I/O), io8_100m_hslv_ft_ms_pd_2v5 (I/O), io8_100m_hslv_ft_ls_2v5 (I/O), io8_100m_hslv_ft_ls_pu_2v5 (I/O), io8_100m_hslv_ft_ls_pd_2v5 (I/O), io8_100m_i2c_ft_1v2 (I/O_open_drain), io8_100m_i2c_ft_pu_1v2 (I/O_open_drain), io8_100m_i2c_ft_pd_1v2 (I/O_open_drain), io8_100m_i2c_ft_1v8 (I/O_open_drain), io8_100m_i2c_ft_pu_1v8 (I/O_open_drain), io8_100m_i2c_ft_pd_1v8 (I/O_open_drain), io8_100m_i2c_ft_3v3 (I/O_open_drain), io8_100m_i2c_ft_pu_3v3 (I/O_open_drain)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
